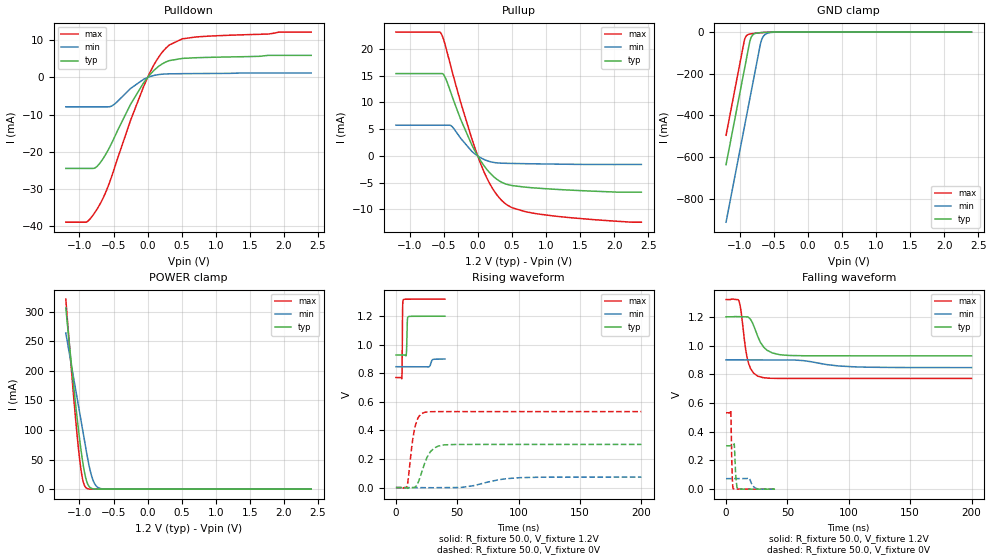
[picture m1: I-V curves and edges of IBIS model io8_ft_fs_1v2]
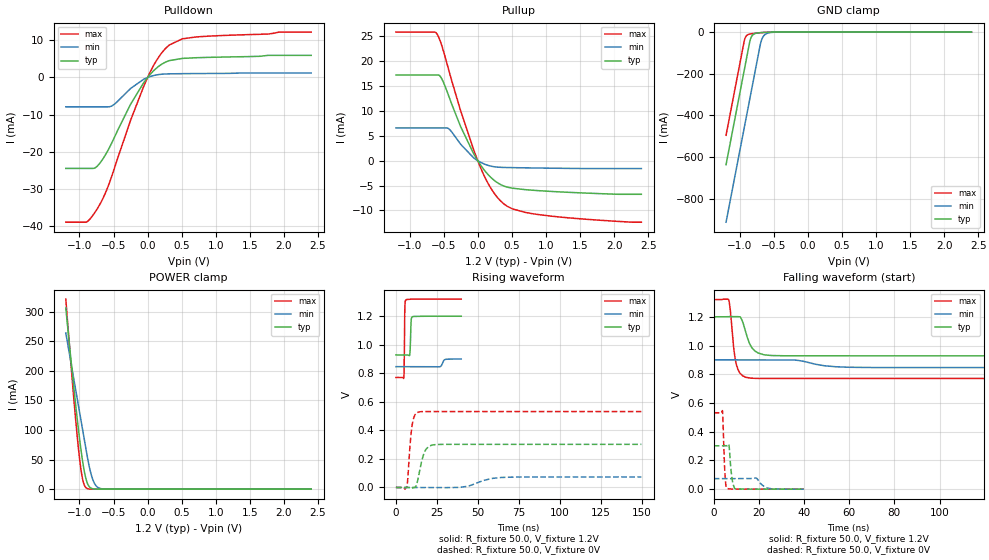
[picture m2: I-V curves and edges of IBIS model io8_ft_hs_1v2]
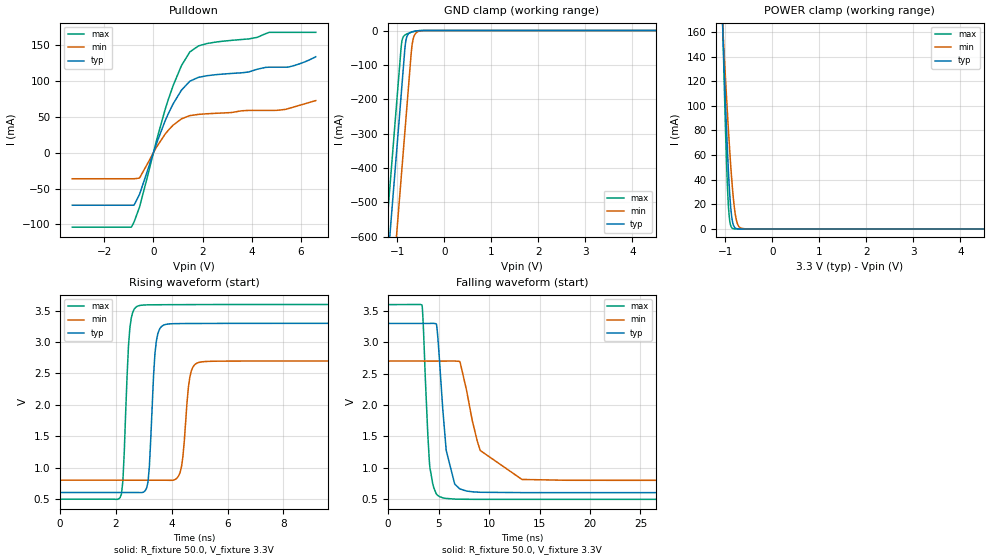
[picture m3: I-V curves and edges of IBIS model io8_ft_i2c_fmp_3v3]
| IBIS file stm32u031_ufqfpn32.ibs
[IBIS ver] 4.2
[File name] stm32u031_ufqfpn32.ibs
[File Rev] 0.2
[Date] 06-05-2024
[Source] Data Created at STMicroelectronics
[Notes]  File originated from ELDO simulations.
[Disclaimer]  This information is for modeling purpose only and is
   not guaranteed. The information is subject to change without
   notice.
[Copyright] Copyright 2024 STMicroelectronics Inc.
|   Component stm32u031_ufqfpn32
[Component] stm32u031_ufqfpn32
[Manufacturer] STMicroelectronics
[Package]
| variable   typ   min   max
R_pkg  0  NA  NA
L_pkg  0  NA  NA
C_pkg  0  NA  NA
[Pin]   signal_name   model_name
1  VDD  power
2  PC14-OSC32_IN  io8_ft_v33
3  PC15-OSC32_OUT  io8_ft
4  PF2-NRST  ioreset_ft_v33
5  VDDA_VREFP  nc
6  PA0-CK_IN  io8_ft_v33
7  PA1  io8_ft_v33
8  PA2  io8_ft_v33
9  PA3  io8_ft
10  PA4  io8_ft
11  PA5  io8_ft
12  PA6  io8_ft_i2c
13  PA7  io8_ft_i2c
14  PB0  io8_ft_i2c
15  PB1  io8_ft
16  VSS  gnd
17  VDD  power
18  PA8  io8_ft
19  PA9  io8_ft_i2c
20  PA10  io8_ft_i2c
21  PA11  io8_ft
22  PA12  io8_ft
23  PA13  io8_ft
24  PA14  io8_ft
25  PA15  io8_ft
26  PB3  io8_ft_i2c
27  PB4  io8_ft_i2c
28  PB5  io8_ft
29  PB6  io8_ft_i2c
30  PB7  io8_ft_i2c
31  PF3-BOOT0  io8_ft_v33
32  VSS  gnd
[Package Model]   459-qfpn-5x5-32-240221
[Pin Mapping]   pulldown_ref   pullup_ref   | Comment
1  nc  vddio
2  gndio  vddio  | Depending on IO usage
| 2  gndio   | Depending on IO usage
3  gndio  vddio  | Depending on IO usage
| 3  gndio   | Depending on IO usage
4  gndio  vddio
5  nc  nc
6  gndio  vddio
7  gndio  vddio
8  gndio  vddio
9  gndio  vddio
10  gndio  vddio
11  gndio  vddio
12  gndio  vddio
13  gndio  vddio
14  gndio  vddio
15  gndio  vddio
16  gndio  nc
17  nc  vddio
18  gndio  vddio
19  gndio  vddio
20  gndio  vddio
21  gndio  vddio
22  gndio  vddio
23  gndio  vddio
24  gndio  vddio
25  gndio  vddio
26  gndio  vddio
27  gndio  vddio
28  gndio  vddio
29  gndio  vddio
30  gndio  vddio
31  gndio  vddio
32  gndio  nc
|[Diff Pin]  inv_pin  vdiff  tdelay_typ  tdelay_min  tdelay_max
|22  21  NA  NA  NA  NA
[Model Selector] io8_ft
io8_ft_ls_1v2   "GPIO - 5V tolerant - 1.2V range - Low speed"
io8_ft_ms_1v2   "GPIO - 5V tolerant - 1.2V range - Med speed"
io8_ft_fs_1v2   "GPIO - 5V tolerant - 1.2V range - Fast speed"
io8_ft_hs_1v2   "GPIO - 5V tolerant - 1.2V range - High speed"
io8_ft_ls_1v8   "GPIO - 5V tolerant - 1.8V range - Low speed"
io8_ft_ms_1v8   "GPIO - 5V tolerant - 1.8V range - Med speed"
io8_ft_fs_1v8   "GPIO - 5V tolerant - 1.8V range - Fast speed"
io8_ft_hs_1v8   "GPIO - 5V tolerant - 1.8V range - High speed"
io8_ft_ls_3v3   "GPIO - 5V tolerant - 3.3V range - Low speed"
io8_ft_ms_3v3   "GPIO - 5V tolerant - 3.3V range - Med speed"
io8_ft_fs_3v3   "GPIO - 5V tolerant - 3.3V range - Fast speed"
io8_ft_hs_3v3   "GPIO - 5V tolerant - 3.3V range - High speed"
[Model Selector] io8_ft_i2c
io8_ft_ls_1v2   "GPIO - 5V tolerant - 1.2V range - Low speed"
io8_ft_ms_1v2   "GPIO - 5V tolerant - 1.2V range - Med speed"
io8_ft_fs_1v2   "GPIO - 5V tolerant - 1.2V range - Fast speed"
io8_ft_hs_1v2   "GPIO - 5V tolerant - 1.2V range - High speed"
io8_ft_ls_1v8   "GPIO - 5V tolerant - 1.8V range - Low speed"
io8_ft_ms_1v8   "GPIO - 5V tolerant - 1.8V range - Med speed"
io8_ft_fs_1v8   "GPIO - 5V tolerant - 1.8V range - Fast speed"
io8_ft_hs_1v8   "GPIO - 5V tolerant - 1.8V range - High speed"
io8_ft_ls_3v3   "GPIO - 5V tolerant - 3.3V range - Low speed"
io8_ft_ms_3v3   "GPIO - 5V tolerant - 3.3V range - Med speed"
io8_ft_fs_3v3   "GPIO - 5V tolerant - 3.3V range - Fast speed"
io8_ft_hs_3v3   "GPIO - 5V tolerant - 3.3V range - High speed"
io8_ft_i2c_ls_1v2   "GPIO I2C open-drain - 5V tolerant - 1.2V range - Low speed"
io8_ft_i2c_ms_1v2   "GPIO I2C open-drain - 5V tolerant - 1.2V range - Med speed"
io8_ft_i2c_fs_1v2   "GPIO I2C open-drain - 5V tolerant - 1.2V range - Fast speed"
io8_ft_i2c_hs_1v2   "GPIO I2C open-drain - 5V tolerant - 1.2V range - High speed"
io8_ft_i2c_ls_1v8   "GPIO I2C open-drain - 5V tolerant - 1.8V range - Low speed"
io8_ft_i2c_ms_1v8   "GPIO I2C open-drain - 5V tolerant - 1.8V range - Med speed"
io8_ft_i2c_fs_1v8   "GPIO I2C open-drain - 5V tolerant - 1.8V range - Fast speed"
io8_ft_i2c_hs_1v8   "GPIO I2C open-drain - 5V tolerant - 1.8V range - High speed"
io8_ft_i2c_ls_3v3   "GPIO I2C open-drain - 5V tolerant - 3.3V range - Low speed"
io8_ft_i2c_ms_3v3   "GPIO I2C open-drain - 5V tolerant - 3.3V range - Med speed"
io8_ft_i2c_fs_3v3   "GPIO I2C open-drain - 5V tolerant - 3.3V range - Fast speed"
io8_ft_i2c_hs_3v3   "GPIO I2C open-drain - 5V tolerant - 3.3V range - High speed"
io8_ft_i2c_fmp_3v3   "GPIO I2C open-drain fm+ - 5V tolerant - 3.3V range"
[Model Selector] io8_ft_v33
io8_ft_v33_ls_1v2   "GPIO_V33 - 5V tolerant - 1.2V range - Low speed"
io8_ft_v33_ms_1v2   "GPIO_V33 - 5V tolerant - 1.2V range - Med speed"
io8_ft_v33_fs_1v2   "GPIO_V33 - 5V tolerant - 1.2V range - Fast speed"
io8_ft_v33_hs_1v2   "GPIO_V33 - 5V tolerant - 1.2V range - High speed"
io8_ft_v33_ls_1v8   "GPIO_V33 - 5V tolerant - 1.8V range - Low speed"
io8_ft_v33_ms_1v8   "GPIO_V33 - 5V tolerant - 1.8V range - Med speed"
io8_ft_v33_fs_1v8   "GPIO_V33 - 5V tolerant - 1.8V range - Fast speed"
io8_ft_v33_hs_1v8   "GPIO_V33 - 5V tolerant - 1.8V range - High speed"
io8_ft_v33_ls_3v3   "GPIO_V33 - 5V tolerant - 3.3V range - Low speed"
io8_ft_v33_ms_3v3   "GPIO_V33 - 5V tolerant - 3.3V range - Med speed"
io8_ft_v33_fs_3v3   "GPIO_V33 - 5V tolerant - 3.3V range - Fast speed"
io8_ft_v33_hs_3v3   "GPIO_V33 - 5V tolerant - 3.3V range - High speed"
[Model Selector] ioreset_ft_v33
ioreset_ft_v33_1v2   "Reset PAD. 5V tolerant. 1.2V range"
ioreset_ft_v33_1v8   "Reset PAD. 5V tolerant. 1.8V range"
ioreset_ft_v33_3v3   "Reset PAD. 5V tolerant. 3.3V range"
[Define Package Model]  459-qfpn-5x5-32-240221
[Manufacturer]  Unknown
[OEM]  Unknown
[Description]  None
[Number Of Pins]  32
[Pin Numbers]
| Pin Num   Terminal Name
6 | PA0-CK_IN
20 | PA10
21 | PA11
22 | PA12
23 | PA13
24 | PA14
25 | PA15
7 | PA1
8 | PA2
9 | PA3
10 | PA4
11 | PA5
12 | PA6
13 | PA7
18 | PA8
19 | PA9
14 | PB0
15 | PB1
26 | PB3
27 | PB4
28 | PB5
29 | PB6
30 | PB7
2 | PC14-OSC32_IN
3 | PC15-OSC32_OUT
4 | PF2-NRST
31 | PF3-BOOT0
17 | VDD
1 | VDD
5 | VDDA_VREFP
32 | VSS
16 | VSS
[Model Data]
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[End Model Data]
[End Package Model]
|End [Component]
| Models and submodels in the file (40): io8_ft_fs_1v2 (I/O), io8_ft_fs_1v8 (I/O), io8_ft_fs_3v3 (I/O), io8_ft_hs_1v2 (I/O), io8_ft_hs_1v8 (I/O), io8_ft_hs_3v3 (I/O), io8_ft_i2c_fmp_3v3 (I/O_open_drain), io8_ft_i2c_fs_1v2 (I/O_open_drain), io8_ft_i2c_fs_1v8 (I/O_open_drain), io8_ft_i2c_fs_3v3 (I/O_open_drain), io8_ft_i2c_hs_1v2 (I/O_open_drain), io8_ft_i2c_hs_1v8 (I/O_open_drain), io8_ft_i2c_hs_3v3 (I/O_open_drain), io8_ft_i2c_ls_1v2 (I/O_open_drain), io8_ft_i2c_ls_1v8 (I/O_open_drain), io8_ft_i2c_ls_3v3 (I/O_open_drain), io8_ft_i2c_ms_1v2 (I/O_open_drain), io8_ft_i2c_ms_1v8 (I/O_open_drain), io8_ft_i2c_ms_3v3 (I/O_open_drain), io8_ft_ls_1v2 (I/O), io8_ft_ls_1v8 (I/O), io8_ft_ls_3v3 (I/O), io8_ft_ms_1v2 (I/O), io8_ft_ms_1v8 (I/O), io8_ft_ms_3v3 (I/O), io8_ft_v33_fs_1v2 (I/O), io8_ft_v33_fs_1v8 (I/O), io8_ft_v33_fs_3v3 (I/O), io8_ft_v33_hs_1v2 (I/O), io8_ft_v33_hs_1v8 (I/O), io8_ft_v33_hs_3v3 (I/O), io8_ft_v33_ls_1v2 (I/O), io8_ft_v33_ls_1v8 (I/O), io8_ft_v33_ls_3v3 (I/O), io8_ft_v33_ms_1v2 (I/O), io8_ft_v33_ms_1v8 (I/O), io8_ft_v33_ms_3v3 (I/O), ioreset_ft_v33_1v2 (I/O_open_drain), ioreset_ft_v33_1v8 (I/O_open_drain), ioreset_ft_v33_3v3 (I/O_open_drain)
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[Model]   io8_ft_fs_1v2
Model_type I/O
Polarity   Non-Inverting
Enable   Active-Low
| CAP_THRESHOLD on pad IOFT is "UDTCAPC" :
| Rising=30.0% of vddiom   Falling=70.0% of vddiom
| C_comp min and max val. don't necessarily correlate with the min and max pvt
| but are the smallest and greatest pad capacitance found.
| var   typ   min   max
C_comp   1.83456pF  1.76047pF  1.83482pF
|C_comp_pullup   1.06365pF  1.01765pF  1.04710pF
|C_comp_pulldown   770.91000fF  742.82001fF  787.72000fF
Vinl = 270.0mV
Vinh = 924.0mV
Vmeas = 600.0mV   | Reference voltage for timing measurements
Cref  = 50.0pF   | Timing specification test load capacitance value
Rref  = 100.0MOhm   | Timing specification test load resistance value
Vref  = 600.0mV   | Timing specification test load voltage
[Model Spec]
| TIME_THRESHOLD on pin ZIV12 is "CMOS" :
| Rising=50.0% of vdd   Falling=50.0% of vdd
Vinl 458.70000mV 364.70000mV 499.70000mV
Vinh 728.30000mV 548.30000mV 792.30000mV
| variable   typ   min   max
[Temperature Range] 25.0 140.0 -40.0
| variable   typ   min   max
[Voltage Range] 1.2V 900.0mV 1.32V
| variable   typ   min   max
[POWER Clamp Reference] 1.2V 900.0mV 1.32V
| variable   typ   min   max
[GND Clamp Reference] 0V 0V 0V
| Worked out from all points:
|   slope of the pulldown table from 0 to 0.18 V, typ, clamps not added: 55.6 ohm
|   slope of the pullup table from 0 to 0.18 V, typ, clamps not added: 56.3 ohm
|   GND clamp passes 1 mA (typ) near -0.61 V on its own axis
|   POWER clamp passes 1 mA (typ) near -0.81 V on its own axis
|   rising waveform, R_fixture 50.0, V_fixture 1.2V: 20-80 % time 436ps typ, 1.3ns min, 278ps max; typ from 0.928 V to 1.2 V
|   falling waveform, R_fixture 50.0, V_fixture 1.2V: 20-80 % time 9.24ns typ, 24.9ns min, 5.52ns max; typ from 1.2 V to 0.928 V
|   rising waveform, R_fixture 50.0, V_fixture 0V: 20-80 % time 8.19ns typ, 23ns min, 4.92ns max; typ from 0 V to 0.302 V
|   falling waveform, R_fixture 50.0, V_fixture 0V: 20-80 % time 1.14ns typ, 2.99ns min, 785ps max; typ from 0.302 V to 0 V
[POWER Clamp]
-1.2V     306.2mA    263.9mA    321.2mA
-1.09V    180mA      191mA      163.4mA
-1.05V    136.9mA    164.5mA    110.9mA
-1.01V    96.55mA    138mA      64.02mA
-960mV    52.29mA    104.9mA    20.68mA
-930mV    31.08mA    85.01mA    7.282mA
-900mV    15.67mA    65.13mA    2.025mA
-850mV    3.417mA    35.2mA     196.2uA
-800mV    570.2uA    14.97mA    18.13uA
-750mV    88.98uA    4.952mA    1.667uA
-680mV    6.495uA    823.9uA    58.96nA
2.4V      0A         0A         0A
[GND Clamp]
-1.2V     -636.9mA   -913.2mA   -495.8mA
-940mV    -194.9mA   -471.2mA   -53.78mA
-920mV    -160.9mA   -437.2mA   -28.06mA
-890mV    -109.9mA   -386.2mA   -14.28mA
-850mV    -43.09mA   -318.2mA   -9.18mA
-820mV    -18.33mA   -267.2mA   -7.516mA
-780mV    -7.695mA   -199.2mA   -5.87mA
-690mV    -2.548mA   -49.42mA   -2.9mA
-660mV    -1.868mA   -24.06mA   -2.112mA
-630mV    -1.326mA   -12.18mA   -1.447mA
-430mV    -19.32uA   -177.8uA   -8.091uA
2.4V      300pA      77.2nA     208.1pA
| variable   typ   min   max
[Pullup Reference] 1.2V 900.0mV 1.32V
| variable   typ   min   max
[Pulldown Reference] 0V 0V 0V
[Pullup]
-1.2V     15.4mA     5.746mA    23.16mA
-540mV    15.4mA     5.746mA    22.96mA
-480mV    14.75mA    5.746mA    20.88mA
-390mV    11.69mA    5.65mA     16.52mA
-250mV    6.833mA    3.296mA    10.02mA
-90mV     2.161mA    908.6uA    3.352mA
30mV      -637.7uA   -235.8uA   -1.032mA
220mV     -3.712mA   -1.175mA   -6.128mA
410mV     -5.232mA   -1.372mA   -8.966mA
510mV     -5.544mA   -1.401mA   -9.708mA
900mV     -6.043mA   -1.482mA   -10.87mA
2.4V      -6.768mA   -1.593mA   -12.38mA
[Pulldown]
-1.2V     -24.47mA   -7.9mA     -38.94mA
-890mV    -24.47mA   -7.9mA     -38.83mA
-720mV    -23.49mA   -7.9mA     -34.76mA
-610mV    -20.54mA   -7.9mA     -30.69mA
-510mV    -17.01mA   -7.49mA    -25.69mA
-250mV    -7.205mA   -2.955mA   -11.53mA
0V        -15fA      0A         0A
160mV     2.97mA     779.9uA    5.417mA
320mV     4.547mA    983.4uA    8.763mA
510mV     5.135mA    1.031mA    10.4mA
700mV     5.311mA    1.057mA    10.88mA
2.4V      5.965mA    1.209mA    12.22mA
[Ramp]
dV/dt_r 181.26153mV/8.18713ns 44.07152mV/22.97907ns 319.20813mV/4.91517ns
dV/dt_f 162.92205mV/9.23981ns 32.18237mV/24.93707ns 329.56896mV/5.51899ns
R_load = 50.0
| Removed startup time: 0s 0s 0s  .
| Removed end time: 39.9ns.
[Rising Waveform]
R_fixture   = 50.0
V_fixture   = 1.2V
V_fixture_min = 900.0mV
V_fixture_max = 1.32V
0s        928.4mV    846.3mV    770.7mV
4.8ns     928.5mV    846.4mV    763.7mV
5.1ns     928.5mV    846.4mV    884.2mV
5.3ns     928.5mV    846.4mV    1.139V
5.5ns     928.5mV    846.4mV    1.282V
6ns       928.5mV    846.4mV    1.315V
8.4ns     926.6mV    846.4mV    1.319V
9.3ns     1.17V      846.4mV    1.319V
9.9ns     1.195V     846.4mV    1.319V
39.9ns    1.2V       899.8mV    1.32V
| Removed startup time: 0s 0s 0s  .
| Removed end time: 199.9ns.
[Falling Waveform]
R_fixture   = 50.0
V_fixture   = 1.2V
V_fixture_min = 900.0mV
V_fixture_max = 1.32V
0s        1.2V       900mV      1.32V
10.2ns    1.202V     900mV      1.316V
12.3ns    1.2V       900mV      1.235V
17.2ns    1.2V       899.9mV    913.2mV
20ns      1.181V     900.7mV    839mV
25.8ns    1.064V     900.4mV    787.2mV
33.3ns    967.8mV    900.2mV    773.7mV
43.6ns    936.4mV    900mV      770.8mV
103.4ns   928.5mV    851.8mV    770.7mV
199.9ns   928.5mV    846.4mV    770.7mV
| Removed startup time: 0s 0s 0s  .
| Removed end time: 199.9ns.
[Rising Waveform]
R_fixture   = 50.0
V_fixture   = 0V
V_fixture_min = 0V
V_fixture_max = 0V
0s        -21.54uV   -19.21uV   -16.71uV
8.9ns     -3.175mV   116.4nV    6.171mV
13.8ns    -309.2uV   111.6nV    344.4mV
15.3ns    1.353mV    38.02nV    417.6mV
18.6ns    45.62mV    -273.8nV   497.4mV
23.5ns    172.6mV    13.25uV    527.2mV
31ns      276mV      -949.2uV   531.9mV
39.7ns    299.2mV    -41.11uV   532mV
101.6ns   302.1mV    69.62mV    532mV
199.9ns   302.1mV    73.45mV    532mV
| Removed startup time: 0s 0s 0s  .
| Removed end time: 39.9ns.
[Falling Waveform]
R_fixture   = 50.0
V_fixture   = 0V
V_fixture_min = 0V
V_fixture_max = 0V
0s        302.1mV    73.47mV    532mV
3.9ns     302.1mV    73.46mV    545.2mV
4.8ns     302mV      73.46mV    149.9mV
5.7ns     301.2mV    73.46mV    4.665mV
6.7ns     313.1mV    73.46mV    1.612mV
7.9ns     95.56mV    73.46mV    813.2uV
9.5ns     1.893mV    73.46mV    702.7uV
18.9ns    336.4uV    77.18mV    91.81uV
25.4ns    142.5uV    1.948mV    17.15uV
39.9ns    20.57uV    72.84uV    2.629uV
[Model]   io8_ft_hs_1v2
Model_type I/O
Polarity   Non-Inverting
Enable   Active-Low
| CAP_THRESHOLD on pad IOFT is "UDTCAPC" :
| Rising=30.0% of vddiom   Falling=70.0% of vddiom
| C_comp min and max val. don't necessarily correlate with the min and max pvt
| but are the smallest and greatest pad capacitance found.
| var   typ   min   max
C_comp   1.83456pF  1.76049pF  1.83488pF
|C_comp_pullup   1.06370pF  1.01770pF  1.04720pF
|C_comp_pulldown   770.86000fF  742.79001fF  787.68000fF
Vinl = 270.0mV
Vinh = 924.0mV
Vmeas = 600.0mV   | Reference voltage for timing measurements
Cref  = 50.0pF   | Timing specification test load capacitance value
Rref  = 100.0MOhm   | Timing specification test load resistance value
Vref  = 600.0mV   | Timing specification test load voltage
[Model Spec]
| TIME_THRESHOLD on pin ZIV12 is "CMOS" :
| Rising=50.0% of vdd   Falling=50.0% of vdd
Vinl 458.70000mV 364.70000mV 499.70000mV
Vinh 728.30000mV 548.30000mV 792.30000mV
| variable   typ   min   max
[Temperature Range] 25.0 140.0 -40.0
| variable   typ   min   max
[Voltage Range] 1.2V 900.0mV 1.32V
| variable   typ   min   max
[POWER Clamp Reference] 1.2V 900.0mV 1.32V
| variable   typ   min   max
[GND Clamp Reference] 0V 0V 0V
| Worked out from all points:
|   slope of the pulldown table from 0 to 0.18 V, typ, clamps not added: 55.6 ohm
|   slope of the pullup table from 0 to 0.18 V, typ, clamps not added: 56.3 ohm
|   GND clamp passes 1 mA (typ) near -0.61 V on its own axis
|   POWER clamp passes 1 mA (typ) near -0.81 V on its own axis
|   rising waveform, R_fixture 50.0, V_fixture 1.2V: 20-80 % time 429ps typ, 1.3ns min, 278ps max; typ from 0.928 V to 1.2 V
|   falling waveform, R_fixture 50.0, V_fixture 1.2V: 20-80 % time 3.78ns typ, 10.4ns min, 2.27ns max; typ from 1.2 V to 0.928 V
|   rising waveform, R_fixture 50.0, V_fixture 0V: 20-80 % time 3.76ns typ, 11.5ns min, 2.21ns max; typ from 0 V to 0.302 V
|   falling waveform, R_fixture 50.0, V_fixture 0V: 20-80 % time 1.15ns typ, 2.99ns min, 786ps max; typ from 0.302 V to 0 V
[POWER Clamp]
-1.2V     306.2mA    263.9mA    321.2mA
-1.09V    180mA      191mA      163.4mA
-1.05V    136.9mA    164.5mA    110.9mA
-1.01V    96.55mA    138mA      64.02mA
-960mV    52.29mA    104.9mA    20.68mA
-930mV    31.08mA    85.01mA    7.282mA
-900mV    15.67mA    65.13mA    2.025mA
-850mV    3.417mA    35.2mA     196.2uA
-800mV    570.2uA    14.97mA    18.13uA
-750mV    88.98uA    4.952mA    1.667uA
-680mV    6.495uA    823.9uA    58.96nA
2.4V      0A         0A         0A
[GND Clamp]
-1.2V     -636.9mA   -913.2mA   -495.8mA
-940mV    -194.9mA   -471.2mA   -53.78mA
-920mV    -160.9mA   -437.2mA   -28.06mA
-890mV    -109.9mA   -386.2mA   -14.28mA
-850mV    -43.09mA   -318.2mA   -9.18mA
-820mV    -18.33mA   -267.2mA   -7.516mA
-780mV    -7.695mA   -199.2mA   -5.87mA
-690mV    -2.548mA   -49.42mA   -2.9mA
-660mV    -1.868mA   -24.06mA   -2.112mA
-630mV    -1.326mA   -12.18mA   -1.447mA
-430mV    -19.32uA   -177.8uA   -8.091uA
2.4V      300pA      77.2nA     208.1pA
| variable   typ   min   max
[Pullup Reference] 1.2V 900.0mV 1.32V
| variable   typ   min   max
[Pulldown Reference] 0V 0V 0V
[Pullup]
-1.2V     17.25mA    6.594mA    25.88mA
-630mV    17.25mA    6.594mA    25.88mA
-600mV    17.25mA    6.594mA    25.56mA
-530mV    16.54mA    6.594mA    23.27mA
-420mV    12.82mA    6.361mA    17.99mA
-250mV    6.833mA    3.302mA    10.02mA
10mV      -217.3uA   -81.33uA   -351.4uA
200mV     -3.465mA   -1.119mA   -5.704mA
390mV     -5.137mA   -1.365mA   -8.762mA
510mV     -5.544mA   -1.401mA   -9.708mA
900mV     -6.043mA   -1.482mA   -10.87mA
2.4V      -6.768mA   -1.593mA   -12.38mA
[Pulldown]
-1.2V     -24.47mA   -7.9mA     -38.94mA
-890mV    -24.47mA   -7.9mA     -38.83mA
-720mV    -23.49mA   -7.9mA     -34.76mA
-610mV    -20.54mA   -7.9mA     -30.69mA
-510mV    -17.01mA   -7.49mA    -25.69mA
-250mV    -7.205mA   -2.955mA   -11.53mA
0V        0A         0A         -16fA
160mV     2.97mA     779.9uA    5.417mA
320mV     4.547mA    983.4uA    8.763mA
510mV     5.135mA    1.031mA    10.4mA
700mV     5.311mA    1.057mA    10.88mA
2.4V      5.965mA    1.209mA    12.22mA
[Ramp]
dV/dt_r 181.26962mV/3.75639ns 44.0861mV/11.48015ns 319.21038mV/2.19825ns
dV/dt_f 162.92582mV/3.78181ns 32.17029mV/10.39666ns 329.57189mV/2.27164ns
R_load = 50.0
| Removed startup time: 0s 0s 0s  .
| Removed end time: 39.9ns.
[Rising Waveform]
R_fixture   = 50.0
V_fixture   = 1.2V
V_fixture_min = 900.0mV
V_fixture_max = 1.32V
0s        928.4mV    846.3mV    770.7mV
4.8ns     928.5mV    846.4mV    764.7mV
5.1ns     928.5mV    846.4mV    885.1mV
5.4ns     928.5mV    846.4mV    1.238V
6ns       928.5mV    846.4mV    1.314V
8.4ns     927mV      846.4mV    1.319V
8.7ns     966.5mV    846.4mV    1.319V
9.3ns     1.17V      846.4mV    1.319V
10ns      1.196V     846.4mV    1.32V
39.9ns    1.2V       899.7mV    1.32V
| Removed startup time: 0s 0s 0s  .
| Removed end time: 149.9ns.
[Falling Waveform]
R_fixture   = 50.0
V_fixture   = 1.2V
V_fixture_min = 900.0mV
V_fixture_max = 1.32V
0s        1.2V       900mV      1.32V
6.7ns     1.201V     900mV      1.316V
8.9ns     1.202V     900mV      972.3mV
9.9ns     1.202V     900mV      874.1mV
11.9ns    1.196V     900mV      802.7mV
14.2ns    1.091V     900mV      778.6mV
18ns      964.8mV    899.9mV    771.7mV
25.5ns    930.4mV    900.4mV    770.7mV
59.8ns    928.5mV    848.8mV    770.7mV
149.9ns   928.5mV    846.4mV    770.7mV
| Removed startup time: 0s 0s 0s  .
| Removed end time: 149.9ns.
[Rising Waveform]
R_fixture   = 50.0
V_fixture   = 0V
V_fixture_min = 0V
V_fixture_max = 0V
0s        -21.52uV   -19.2uV    -16.69uV
6.6ns     92.12nV    212.2nV    3.073mV
7.2ns     29.66uV    184.2nV    52.81mV
9.7ns     -4.874mV   167.6nV    423.4mV
12.1ns    5.843mV    200.8nV    515.7mV
13.9ns    83.49mV    113.1nV    529.1mV
16.9ns    232.8mV    -27.83nV   531.8mV
22ns      297.2mV    2.952uV    532mV
64.7ns    302.1mV    70.19mV    532mV
149.9ns   302.1mV    73.48mV    532mV
| Removed startup time: 0s 0s 0s  .
| Removed end time: 39.9ns.
[Falling Waveform]
R_fixture   = 50.0
V_fixture   = 0V
V_fixture_min = 0V
V_fixture_max = 0V
0s        302.1mV    73.47mV    532mV
3.9ns     302.1mV    73.46mV    542.4mV
4.8ns     302mV      73.46mV    149.8mV
5.3ns     301.8mV    73.46mV    34.07mV
5.7ns     301.4mV    73.46mV    5.584mV
6.7ns     311.1mV    73.46mV    2.56mV
7.8ns     107.8mV    73.46mV    976.5uV
9.2ns     5.754mV    73.46mV    394.7uV
26ns      4.46uV     1.169mV    -6.739uV
39.9ns    -2.54uV    150.5uV    -6.345uV
[Model]   io8_ft_i2c_fmp_3v3
Model_type I/O_open_drain
Polarity   Non-Inverting
Enable   Active-Low
| CAP_THRESHOLD on pad IOFT is "UDTCAPC" :
| Rising=30.0% of vddiom   Falling=70.0% of vddiom
| C_comp min and max val. don't necessarily correlate with the min and max pvt
| but are the smallest and greatest pad capacitance found.
| var   typ   min   max
C_comp   2.58496pF  2.53515pF  2.60374pF
|C_comp_pulldown   2.58496pF  2.53515pF  2.60374pF
Vinl = 1.35V
Vinh = 1.8V
Vmeas = 1.65V   | Reference voltage for timing measurements
Cref  = 50.0pF   | Timing specification test load capacitance value
Rref  = 1.0MOhm   | Timing specification test load resistance value
Vref  = 1.815V   | Timing specification test load voltage
[Model Spec]
| TIME_THRESHOLD on pin ZIV12 is "CMOS" :
| Rising=50.0% of vdd   Falling=50.0% of vdd
Vinl 1.34770V 1.11370V 1.44970V
Vinh 1.77530V 1.49530V 1.90330V
| variable   typ   min   max
[Temperature Range] 25.0 125.0 -40.0
| variable   typ   min   max
[Voltage Range] 3.3V 2.7V 3.6V
| variable   typ   min   max
[POWER Clamp Reference] 3.3V 2.7V 3.6V
| variable   typ   min   max
[GND Clamp Reference] 0V 0V 0V
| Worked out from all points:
|   slope of the pulldown table from 0 to 0.495 V, typ, clamps not added: 10.9 ohm
|   GND clamp passes 1 mA (typ) near -0.58 V on its own axis
|   POWER clamp passes 1 mA (typ) near -0.80 V on its own axis
|   rising waveform, R_fixture 50.0, V_fixture 3.3V: 20-80 % time 178ps typ, 208ps min, 172ps max; typ from 0.603 V to 3.3 V
|   falling waveform, R_fixture 50.0, V_fixture 3.3V: 20-80 % time 896ps typ, 2.33ns min, 522ps max; typ from 3.3 V to 0.603 V
[POWER Clamp]
-3.3V     3.015A     2.054A     3.978A
-1.06V    166.8mA    167.3mA    172.4mA
-1.05V    156mA      159.9mA    156.7mA
-980mV    85.12mA    110.1mA    59.21mA
-940mV    50.68mA    83.63mA    21.78mA
-920mV    36.19mA    71.13mA    10.91mA
-890mV    19.13mA    53.62mA    3.147mA
-840mV    4.466mA    28.96mA    309.8uA
-790mV    763.7uA    12.17mA    28.67uA
-740mV    119.7uA    3.892mA    2.636uA
-560mV    142.6nA    28.01uA    519.9pA
6.6V      0A         0A         0A
[GND Clamp]
-3.3V     -4.231A    -4.473A    -4.091A
-1.25V    -746.3mA   -988.1mA   -606.2mA
-930mV    -202.3mA   -444.1mA   -62.21mA
-910mV    -168.3mA   -410.1mA   -35.02mA
-840mV    -49.53mA   -291.1mA   -13.04mA
-820mV    -28.87mA   -257.1mA   -11.41mA
-780mV    -12.16mA   -189.1mA   -8.87mA
-720mV    -5.351mA   -87.09mA   -5.703mA
-690mV    -3.9mA     -43.52mA   -4.338mA
-650mV    -2.532mA   -17.76mA   -2.784mA
-480mV    -113.2uA   -482.1uA   -69.15uA
6.6V      840.8pA    92.11nA    588.9pA
| variable   typ   min   max
[Pullup Reference] 3.3V 2.7V 3.6V
| variable   typ   min   max
[Pulldown Reference] 0V 0V 0V
[Pulldown]
-3.3V     -73.23mA   -36.43mA   -103.7mA
-890mV    -73.23mA   -36.43mA   -103.1mA
-790mV    -73.08mA   -36.43mA   -96.56mA
-570mV    -58.43mA   -35.54mA   -76.22mA
120mV     12.17mA    7.266mA    16.35mA
600mV     53.75mA    30.83mA    73.34mA
1.14V     86.74mA    46.88mA    120.9mA
1.48V     99.14mA    51.31mA    139.9mA
2.17V     106.7mA    53.87mA    151.5mA
4.71V     118.6mA    58.52mA    167.1mA
5.5V      118.8mA    61.2mA     167.1mA
6.6V      133.1mA    72.2mA     167.1mA
[Ramp]
dV/dt_r 1.61843V/174.41251ps 1.14071V/206.39789ps 1.86269V/168.33494ps
dV/dt_f 1.61846V/796.60522ps 1.14076V/1.69774ns 1.86272V/521.88482ps
R_load = 50.0
| Removed startup time: 0s 0s 0s  .
| Removed end time: 19.75ns.
[Rising Waveform]
R_fixture   = 50.0
V_fixture   = 3.3V
V_fixture_min = 2.7V
V_fixture_max = 3.6V
0s        602.6mV    798.7mV    495.5mV
2.15ns    602.5mV    798.7mV    522.1mV
2.5ns     602.5mV    798.7mV    3.227V
2.8ns     602mV      798.6mV    3.578V
3.15ns    767.9mV    798.6mV    3.594V
3.4ns     2.823V     798.6mV    3.596V
3.75ns    3.278V     798mV      3.597V
4.3ns     3.296V     922.6mV    3.598V
5ns       3.297V     2.679V     3.599V
19.75ns   3.3V       2.7V       3.6V
| Removed startup time: 0s 0s 0s  .
| Removed end time: 39.775ns.
[Falling Waveform]
R_fixture   = 50.0
V_fixture   = 3.3V
V_fixture_min = 2.7V
V_fixture_max = 3.6V
0s        3.3V       2.7V       3.6V
3.365ns   3.3V       2.7V       3.588V
4.13ns    3.3V       2.7V       1.023V
4.795ns   3.283V     2.7V       580.3mV
5.125ns   2.632V     2.7V       537.2mV
5.755ns   1.278V     2.7V       509.6mV
7.13ns    660.5mV    2.685V     497.4mV
9.13ns    608.1mV    1.274V     495.6mV
13.26ns   602.6mV    812.4mV    495.5mV
39.78ns   602.6mV    798.7mV    495.5mV
